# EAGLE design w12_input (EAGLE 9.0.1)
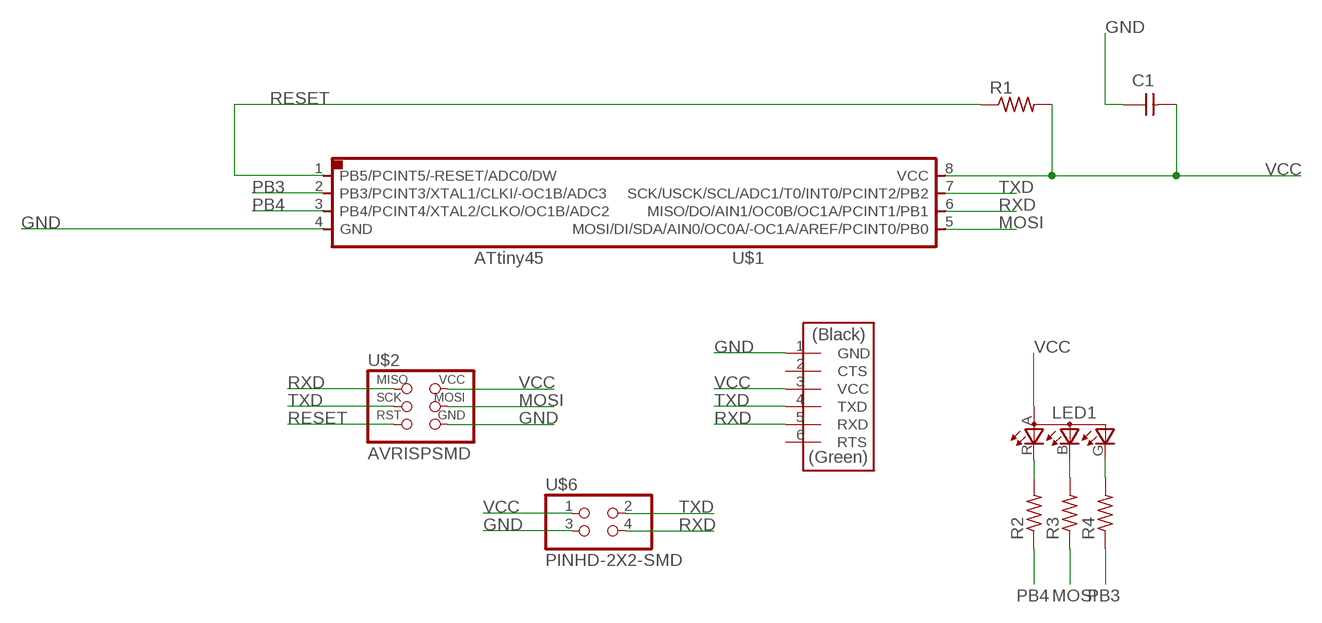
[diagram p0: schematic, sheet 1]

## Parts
C1  CAP-UNPOLARIZEDFAB  [C1206FAB]
LED1  LEDRGBOLD  [P-LCC-4-3]
R1  RES-US1206FAB  [R1206FAB]
R2  RES-US1206FAB  [R1206FAB]
R3  RES-US1206FAB  [R1206FAB]
R4  RES-US1206FAB  [R1206FAB]
U$1  ATTINY45SI  [SOIC8]
U$2  AVRISPSMD  [2X03SMD]
U$3  FTDI-SMD-HEADER  [1X06SMD]
U$6  PINHD-2X2-SMD  [2X02SMD]

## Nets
GND: C1.1 U$1.4(GND) U$2.6(GND) U$3.1(GND) U$6.3
MOSI: R3.1 U$1.5(MOSI/DI/SDA/AIN0/OC0A/-OC1A/AREF/PCINT0/PB0) U$2.4(MOSI)
N$1: LED1.R(CRED) R2.2
N$2: LED1.B(CBLUE) R3.2
N$3: LED1.G(CGREEN) R4.2
PB3: R4.1 U$1.2(PB3/PCINT3/XTAL1/CLKI/-OC1B/ADC3)
PB4: R2.1 U$1.3(PB4/PCINT4/XTAL2/CLKO/OC1B/ADC2)
RESET: R1.1 U$1.1(PB5/PCINT5/-RESET/ADC0/DW) U$2.5(RST)
RXD: U$1.6(MISO/DO/AIN1/OC0B/OC1A/PCINT1/PB1) U$2.1(MISO) U$3.5(RXD) U$6.4
TXD: U$1.7(SCK/USCK/SCL/ADC1/T0/INT0/PCINT2/PB2) U$2.3(SCK) U$3.4(TXD) U$6.2
VCC: C1.2 LED1.A(A2) R1.2 U$1.8(VCC) U$2.2(VCC) U$3.3(VCC) U$6.1
Unconnected: U$3.2(CTS) U$3.6(RTS)

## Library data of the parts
C1 = fab:CAP-UNPOLARIZED
LED1 = fab:LEDRGBOLD: OSRAM Hyper Multi TOPLED® Hyper-Bright LED LATB T686 Source: http://www.osram.convergy.de/
R1-R4 = fab:RES-US: Resistor (US Symbol)
U$1 = fab:ATTINY45
U$2 = fab:AVRISP
U$3 = fab:FTDI-SMD-HEADER
U$6 = fab:PINHD-2X2-SMD

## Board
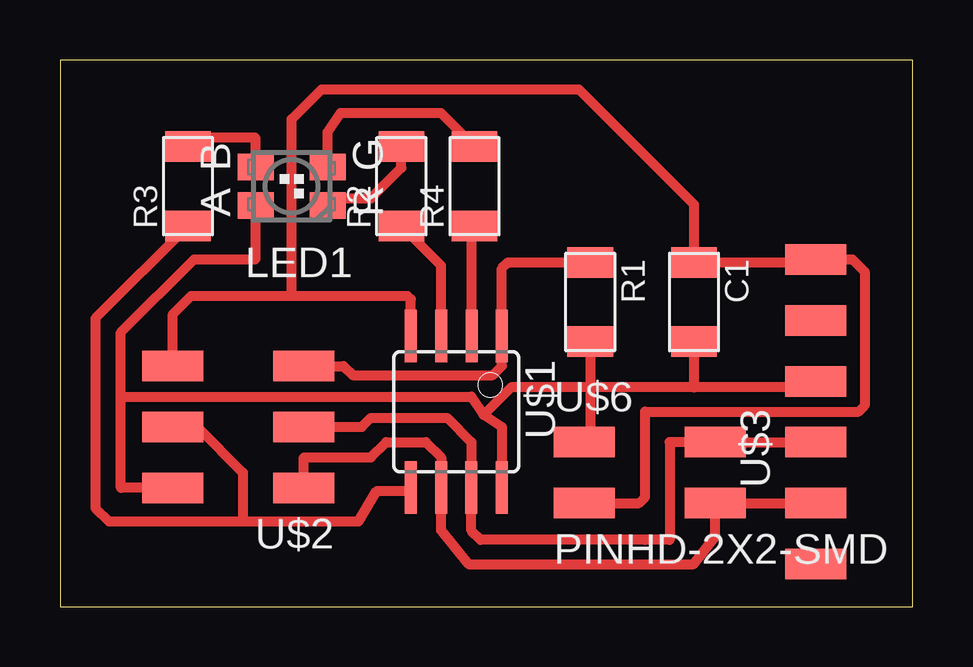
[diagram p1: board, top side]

Size 35.54 x 22.78 mm. Coordinates in mm from the lower left corner, seen from the top.
Outline: 0,0 35.54,0 35.54,22.78 0,22.78 0,0
Copper layers (1*16): Top 0.035mm / dielectric 1.5mm / Bottom 0.035mm
Design rules "default": minimum track width 6mil, minimum drill 0.35mm, track to track 6mil, track to pad 6mil, pad to pad 6mil, via to via 6mil, smd to smd 6mil, copper to edge 40mil, drill to drill 6mil, minimum pad ring 10mil, minimum via ring 8mil, stop-mask expansion 4mil, vias tented up to drill 0mil, thermal gap 10mil

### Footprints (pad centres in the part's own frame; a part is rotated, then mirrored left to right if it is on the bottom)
C1206FAB = smd 1.27 x 1.905: 1 -1.651,0; 2 1.651,0
P-LCC-4-3 = smd 1.1 x 1.5: A -0.8,1.5; B 0.8,1.5; G 0.8,-1.5; R -0.8,-1.5
R1206FAB = smd 1.27 x 1.905: 1 -1.651,0; 2 1.651,0
SOIC8 = smd 0.5 x 2.2: 1 -1.905,-3.154; 2 -0.645,-3.154; 3 0.625,-3.154; 4 1.895,-3.154; 5 1.905,3.154; 6 0.635,3.154; 7 -0.635,3.154; 8 -1.905,3.154
2X03SMD = smd 2.54 x 1.27: 1 -2.54,2.54; 2 2.92,2.54; 3 -2.54,0; 4 2.92,0; 5 -2.54,-2.54; 6 2.92,-2.54
1X06SMD = smd 2.54 x 1.27: 1 0,6.35; 2 0,3.81; 3 0,1.27; 4 0,-1.27; 5 0,-3.81; 6 0,-6.35
2X02SMD = smd 2.54 x 1.27: 1 -2.54,1.27; 2 2.92,1.27; 3 -2.54,-1.27; 4 2.92,-1.27

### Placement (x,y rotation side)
C1  26.42,12.7 270 top
LED1  9.65,17.53 90 top
R1  22.1,12.7 270 top
R2  14.22,17.53 90 top
R3  5.33,17.53 90 top
R4  17.27,17.53 90 top
U$1  16.51,8.13 180 top
U$2  7.62,7.49 180 top
U$3  31.5,8.13 0 top
U$6  24.38,5.59 0 top

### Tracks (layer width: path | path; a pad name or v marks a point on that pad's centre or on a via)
GND
  Top 0.406: U$1.4 14.62,12.82 14.48,12.95 9.65,12.95 | U$2.6 4.7,12.19 5.46,12.95 9.65,12.95 | U$6.3 24.13,4.32 24.38,4.57 24.38,8.13 33.27,8.13 33.53,8.38 33.53,13.97 33.02,14.48 U$3.1 31.37,14.35 C1.1 | 9.65,12.95 9.65,20.32 10.9,21.56 21.62,21.56 26.42,16.76 C1.1 | 26.42,14.99 C1.1
MOSI
  Top 0.406: U$2.4 5.72,7.49 7.62,5.59 7.62,3.56 | 7.62,3.56 12.45,3.56 13.21,4.83 14.6,4.83 U$1.5 | R3.1 1.47,12.01 1.47,4.12 2.03,3.56 7.62,3.56
N$1
  Top 0.406: R2.2 14.22,18.29 12.95,17.02 11.44,17.02 LED1.R
N$2
  Top 0.406: 5.46,19.3 R3.2 5.72,19.56 8.13,19.56 8.13,18.35 LED1.B
N$3
  Top 0.406: LED1.G 11.15,19.79 11.68,20.57 15.88,20.57 R4.2
PB3
  Top 0.406: U$1.2 17.16,15.76 R4.1
PB4
  Top 0.406: U$1.3 15.88,14.21 R2.1
RESET
  Top 0.406: U$2.5 11.81,10.03 12.19,9.65 18.03,9.65 18.41,10.03 U$1.1 18.41,14.1 18.67,14.35 R1.1
RXD
  Top 0.406: U$3.5 U$6.4 27.3,2.92 26.42,1.78 17.02,1.78 15.88,3.17 U$1.6 15.88,6.22 15.24,6.86 13.59,6.86 12.95,6.22 10.16,6.22 U$2.1
TXD
  Top 0.406: U$3.4 U$6.2 25.4,6.86 25.4,2.79 24.38,2.79 17.53,2.79 17.15,3.17 U$1.7 17.15,6.86 16.13,7.87 12.95,7.87 12.57,7.49 U$2.3
VCC
  Top 0.406: U$2.2 2.54,4.95 2.54,8.76 | 2.54,8.76 17.15,8.76 17.65,8 | 17.65,8 18.41,7.49 U$1.8 | U$3.3 31.24,9.14 26.42,9.14 | 17.65,8 18.8,9.14 22.1,9.14 | 26.42,9.14 22.1,9.14 | R1.2 22.1,9.14 | 22.1,9.14 22.1,7.11 U$6.1 | C1.2 26.42,9.14 | 2.54,8.76 2.54,11.43 5.59,14.48 8.13,14.48 8.15,14.5 LED1.A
